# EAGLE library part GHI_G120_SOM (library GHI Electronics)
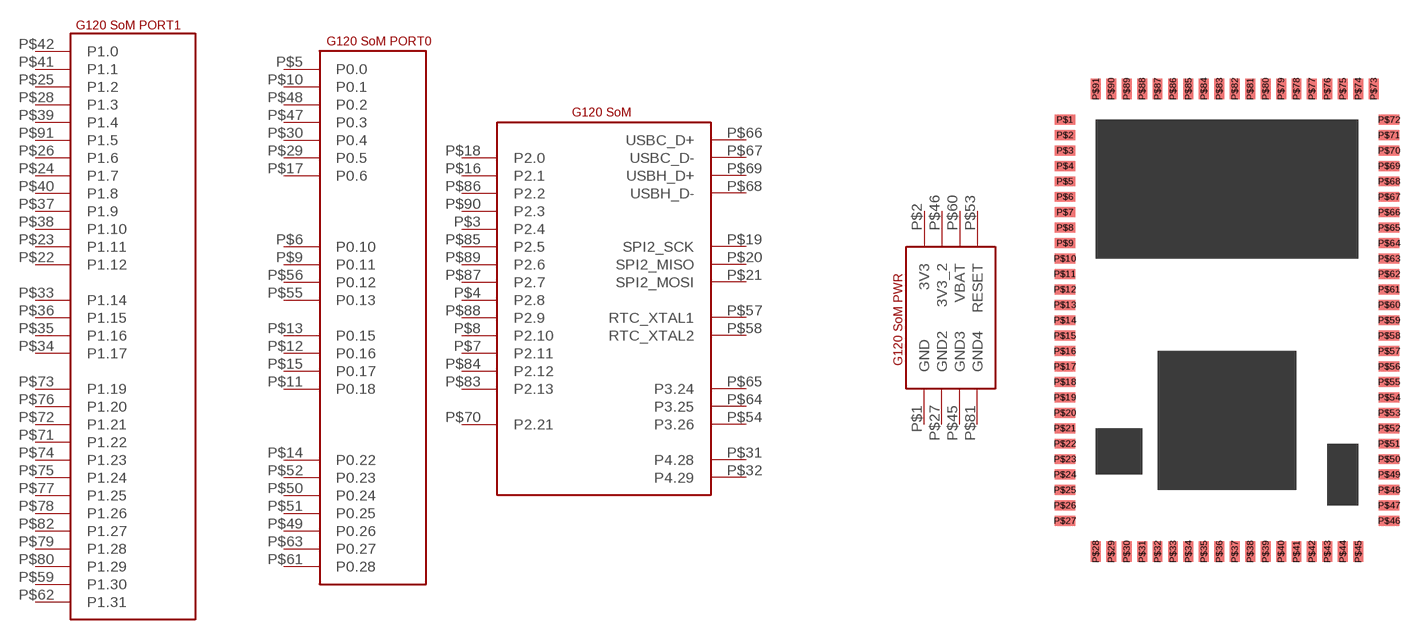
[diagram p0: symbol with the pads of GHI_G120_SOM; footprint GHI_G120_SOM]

Designator prefix -; gates G$1=GHI_G120 G$2=GHI_G120_PORT0 G$3=GHI_G120_PORT1 G$4=GHI_G120_PWR

## GHI_G120_SOM  [GHI_G120_SOM]
P$1  G$4:GND
P$2  G$4:3V3
P$3  G$1:P2.4
P$4  G$1:P2.8
P$5  G$2:P0.0
P$6  G$2:P0.10
P$7  G$1:P2.11
P$8  G$1:P2.10
P$9  G$2:P0.11
P$10  G$2:P0.1
P$11  G$2:P0.18
P$12  G$2:P0.16
P$13  G$2:P0.15
P$14  G$2:P0.22
P$15  G$2:P0.17
P$16  G$1:P2.1
P$17  G$2:P0.6
P$18  G$1:P2.0
P$19  G$1:SPI2_SCK
P$20  G$1:SPI2_MISO
P$21  G$1:SPI2_MOSI
P$22  G$3:P1.12
P$23  G$3:P1.11
P$24  G$3:P1.7
P$25  G$3:P1.2
P$26  G$3:P1.6
P$27  G$4:GND2
P$28  G$3:P1.3
P$29  G$2:P0.5
P$30  G$2:P0.4
P$31  G$1:P4.28
P$32  G$1:P4.29
P$33  G$3:P1.14
P$34  G$3:P1.17
P$35  G$3:P1.16
P$36  G$3:P1.15
P$37  G$3:P1.9
P$38  G$3:P1.10
P$39  G$3:P1.4
P$40  G$3:P1.8
P$41  G$3:P1.1
P$42  G$3:P1.0
P$45  G$4:GND3
P$46  G$4:3V3_2
P$47  G$2:P0.3
P$48  G$2:P0.2
P$49  G$2:P0.26
P$50  G$2:P0.24
P$51  G$2:P0.25
P$52  G$2:P0.23
P$53  G$4:RESET
P$54  G$1:P3.26
P$55  G$2:P0.13
P$56  G$2:P0.12
P$57  G$1:RTC_XTAL1
P$58  G$1:RTC_XTAL2
P$59  G$3:P1.30
P$60  G$4:VBAT
P$61  G$2:P0.28
P$62  G$3:P1.31
P$63  G$2:P0.27
P$64  G$1:P3.25
P$65  G$1:P3.24
P$66  G$1:USBC_D+
P$67  G$1:USBC_D-
P$68  G$1:USBH_D-
P$69  G$1:USBH_D+
P$70  G$1:P2.21
P$71  G$3:P1.22
P$72  G$3:P1.21
P$73  G$3:P1.19
P$74  G$3:P1.23
P$75  G$3:P1.24
P$76  G$3:P1.20
P$77  G$3:P1.25
P$78  G$3:P1.26
P$79  G$3:P1.28
P$80  G$3:P1.29
P$81  G$4:GND4
P$82  G$3:P1.27
P$83  G$1:P2.13
P$84  G$1:P2.12
P$85  G$1:P2.5
P$86  G$1:P2.2
P$87  G$1:P2.7
P$88  G$1:P2.9
P$89  G$1:P2.6
P$90  G$1:P2.3
P$91  G$3:P1.5

## Footprint GHI_G120_SOM (pad centres in mm)
smd 1.676 x 0.813: P$1 -13.97,15.24; P$2 -13.97,13.97; P$3 -13.97,12.7; P$4 -13.97,11.43; P$5 -13.97,10.16; P$6 -13.97,8.89; P$7 -13.97,7.62; P$8 -13.97,6.35; P$9 -13.97,5.08; P$10 -13.97,3.81; P$11 -13.97,2.54; P$12 -13.97,1.27; P$13 -13.97,0; P$14 -13.97,-1.27; P$15 -13.97,-2.54; P$16 -13.97,-3.81; P$17 -13.97,-5.08; P$18 -13.97,-6.35; P$19 -13.97,-7.62; P$20 -13.97,-8.89; P$21 -13.97,-10.16; P$22 -13.97,-11.43; P$23 -13.97,-12.7; P$24 -13.97,-13.97; P$25 -13.97,-15.24; P$26 -13.97,-16.51; P$27 -13.97,-17.78; P$46 12.7,-17.78; P$47 12.7,-16.51; P$48 12.7,-15.24; P$49 12.7,-13.97; P$50 12.7,-12.7; P$51 12.7,-11.43; P$52 12.7,-10.16; P$53 12.7,-8.89; P$54 12.7,-7.62; P$55 12.7,-6.35; P$56 12.7,-5.08; P$57 12.7,-3.81; P$58 12.7,-2.54; P$59 12.7,-1.27; P$60 12.7,0; P$61 12.7,1.27; P$62 12.7,2.54; P$63 12.7,3.81; P$64 12.7,5.08; P$65 12.7,6.35; P$66 12.7,7.62; P$67 12.7,8.89; P$68 12.7,10.16; P$69 12.7,11.43; P$70 12.7,12.7; P$71 12.7,13.97; P$72 12.7,15.24
smd 0.813 x 1.676: P$28 -11.43,-20.32; P$29 -10.16,-20.32; P$30 -8.89,-20.32; P$31 -7.62,-20.32; P$32 -6.35,-20.32; P$33 -5.08,-20.32; P$34 -3.81,-20.32; P$35 -2.54,-20.32; P$36 -1.27,-20.32; P$37 0,-20.32; P$38 1.27,-20.32; P$39 2.54,-20.32; P$40 3.81,-20.32; P$41 5.08,-20.32; P$42 6.35,-20.32; P$43 7.62,-20.32; P$44 8.89,-20.32; P$45 10.16,-20.32; P$73 11.43,17.78; P$74 10.16,17.78; P$75 8.89,17.78; P$76 7.62,17.78; P$77 6.35,17.78; P$78 5.08,17.78; P$79 3.81,17.78; P$80 2.54,17.78; P$81 1.27,17.78; P$82 0,17.78; P$83 -1.27,17.78; P$84 -2.54,17.78; P$85 -3.81,17.78; P$86 -5.08,17.78; P$87 -6.35,17.78; P$88 -7.62,17.78; P$89 -8.89,17.78; P$90 -10.16,17.78; P$91 -11.43,17.78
